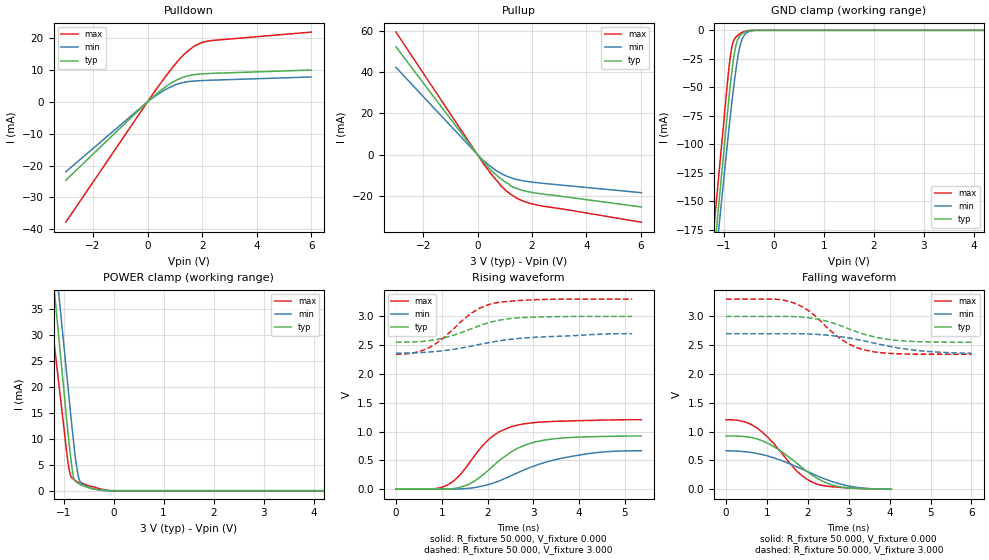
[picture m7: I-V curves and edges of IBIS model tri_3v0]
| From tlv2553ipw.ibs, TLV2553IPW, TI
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[Model]   tri_3v0
Model_type 3-state
Vref=0.000E+00
Rref=5.000E+06
Cref=3.000E-11
Vmeas=1.500E+00
C_comp  2.00000pF 2.00000pF 2.00000pF
[Model Spec]
[Voltage Range]   3.000E+00   2.700E+00   3.300E+00
[POWER Clamp Reference]   3.000E+00   2.700E+00   3.300E+00
[GND Clamp Reference]   0.000E+00   0.000E+00   0.000E+00
[Pullup Reference]   3.000E+00   2.700E+00   3.300E+00
[Pulldown Reference]   0.000E+00   0.000E+00   0.000E+00
[Temperature Range]   25   105   -40
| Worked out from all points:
|   slope of the pulldown table from 0 to 0.45 V, typ, clamps not added: 136 ohm
|   slope of the pullup table from 0 to 0.45 V, typ, clamps not added: 65.4 ohm
|   GND clamp passes 1 mA (typ) near -0.55 V on its own axis
|   POWER clamp passes 1 mA (typ) near -0.63 V on its own axis
|   rising waveform, R_fixture 50.000, V_fixture 0.000: 20-80 % time 940ps typ, 1.37ns min, 801ps max; typ from 0 V to 0.923 V
|   falling waveform, R_fixture 50.000, V_fixture 0.000: 20-80 % time 1.07ns typ, 1.38ns min, 921ps max; typ from 0.923 V to 0 V
|   rising waveform, R_fixture 50.000, V_fixture 3.000: 20-80 % time 1ns typ, 1.66ns min, 875ps max; typ from 2.55 V to 3 V
|   falling waveform, R_fixture 50.000, V_fixture 3.000: 20-80 % time 1.15ns typ, 1.49ns min, 967ps max; typ from 3 V to 2.55 V
[GND Clamp]
-3V       -1.034A    -997mA     -1.021A
-1.02V    -115.8mA   -139.5mA   -89.71mA
-900mV    -60.8mA    -87.77mA   -34.5mA
-840mV    -36.94mA   -63.96mA   -14.96mA
-780mV    -18.33mA   -42.13mA   -7.249mA
-740mV    -10.44mA   -29.3mA    -5.162mA
-700mV    -6.262mA   -18.75mA   -3.735mA
-660mV    -3.894mA   -11.04mA   -2.408mA
-600mV    -2.044mA   -5.019mA   -1.167mA
-520mV    -600uA     -1.482mA   -252.3uA
-360mV    -1.046uA   -1.184uA   225.7nA
6V        7.322uA    8.286uA    1.354uA
[Power Clamp]
-3V       220.1mA    223mA      179.4mA
-1.02V    22.01mA    30.54mA    14.37mA
-940mV    13.96mA    22.74mA    7.642mA
-900mV    10.06mA    18.87mA    4.633mA
-860mV    6.707mA    14.94mA    2.904mA
-800mV    2.461mA    9.488mA    2.192mA
-760mV    1.787mA    6.121mA    1.893mA
-700mV    1.35mA     2.577mA    1.58mA
-640mV    1.034mA    1.342mA    1.518mA
-420mV    364.3uA    393uA      767.6uA
-20mV     -36.92nA   -14.5uA    -60.08uA
6.02V     -36.92nA   -14.5uA    -60.08uA
[Pullup]
-3V       52.2mA     42.27mA    59.31mA
80mV      -1.343mA   -1.08mA    -1.623mA
520mV     -7.83mA    -6.138mA   -9.632mA
820mV     -11.32mA   -8.737mA   -14.21mA
840mV     -11.52mA   -8.892mA   -14.91mA
1.18V     -14.46mA   -10.95mA   -18.84mA
1.22V     -15.12mA   -11.14mA   -19.18mA
1.56V     -16.93mA   -12.35mA   -21.81mA
2.16V     -18.6mA    -13.51mA   -24.31mA
6.02V     -25.31mA   -18.39mA   -32.67mA
[Pulldown]
-3V       -24.61mA   -21.95mA   -37.74mA
60mV      491.2uA    434.4uA    757.3uA
500mV     3.658mA    3.035mA    6.079mA
920mV     6.125mA    4.948mA    10.8mA
1.36V     7.845mA    6.123mA    15.09mA
1.5V      8.178mA    6.319mA    16.05mA
1.72V     8.508mA    6.504mA    17.49mA
1.9V      8.671mA    6.602mA    18.24mA
2.32V     8.883mA    6.754mA    19.16mA
6V        9.937mA    7.768mA    21.83mA
[Rising Waveform]
R_fixture = 50.000
V_fixture = 0.000
V_fixture_min = 0.000
V_fixture_max = 0.000
|  time   V(typ)   V(min)   V(max)
0s        -258.1uV   205.5uV    1.835mV
800ps     -207uV     257uV      4.539mV
1.12ns    1.532mV    -175.9uV   70.3mV
1.36ns    24.77mV    2.36mV     215.1mV
1.6ns     89.51mV    15.4mV     452.8mV
2.04ns    344.8mV    84.11mV    872mV
2.56ns    666.7mV    248.9mV    1.094V
3.04ns    818.6mV    407.9mV    1.157V
3.76ns    895.3mV    558mV      1.184V
5.36ns    922.6mV    666.2mV    1.206V
[Falling Waveform]
R_fixture = 50.000
V_fixture = 0.000
V_fixture_min = 0.000
V_fixture_max = 0.000
|  time   V(typ)   V(min)   V(max)
0s        922.6mV    666.2mV    1.206V
440ps     914.2mV    651.6mV    1.172V
760ps     871.5mV    619.5mV    1.06V
1.2ns     724.4mV    535.2mV    763.3mV
1.76ns    433.1mV    379.2mV    294.9mV
2.16ns    218.5mV    252.3mV    105.6mV
2.48ns    101.8mV    159.4mV    50.5mV
2.8ns     38.69mV    87.67mV    30.83mV
3.32ns    9.125mV    20.46mV    11.18mV
4.04ns    -258.1uV   205.5uV    1.835mV
[Rising Waveform]
R_fixture = 50.000
V_fixture = 3.000
V_fixture_min = 2.700
V_fixture_max = 3.300
|  time   V(typ)   V(min)   V(max)
0s        2.552V     2.362V     2.344V
400ps     2.558V     2.368V     2.369V
760ps     2.583V     2.385V     2.473V
1.04ns    2.626V     2.406V     2.628V
1.64ns    2.784V     2.484V     3.052V
1.92ns    2.865V     2.529V     3.175V
2.16ns    2.918V     2.563V     3.233V
2.52ns    2.966V     2.605V     3.266V
2.88ns    2.984V     2.63V      3.285V
5.16ns    3V         2.7V       3.302V
[Falling Waveform]
R_fixture = 50.000
V_fixture = 3.000
V_fixture_min = 2.700
V_fixture_max = 3.300
|  time   V(typ)   V(min)   V(max)
0s        3V         2.7V       3.302V
1.16ns    3V         2.7V       3.302V
1.68ns    2.997V     2.7V       3.227V
2.04ns    2.974V     2.694V     3.09V
2.6ns     2.889V     2.666V     2.723V
2.88ns    2.818V     2.64V      2.573V
3.12ns    2.753V     2.612V     2.482V
3.44ns    2.678V     2.566V     2.409V
4.44ns    2.57V      2.429V     2.347V
6ns       2.552V     2.362V     2.344V
[Ramp]
| variable typ min max
dV/dt_r 553.650m/1.01708n 399.243m/1.52094n 722.983m/847.875p
dV/dt_f 267.306m/1.13960n 349.048m/1.48000n 576.118m/956.962p
R_load = 50.0000Ohms
